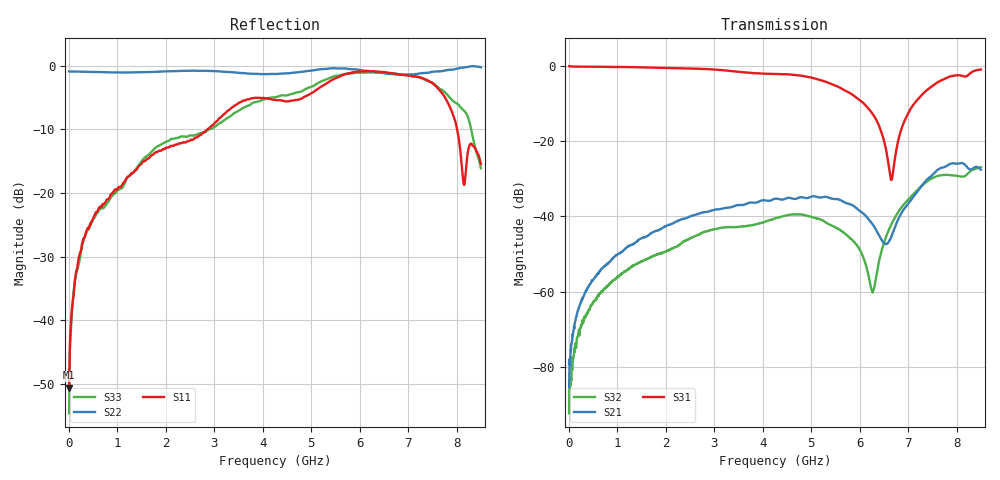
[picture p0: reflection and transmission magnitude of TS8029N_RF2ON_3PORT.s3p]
!Created with skrf (http://scikit-rf.org).
# GHz S RI R 50.0
!freq ReS11 ImS11 ReS12 ImS12 ReS13 ImS13
! ReS21 ImS21 ReS22 ImS22 ReS23 ImS23
! ReS31 ImS31 ReS32 ImS32 ReS33 ImS33
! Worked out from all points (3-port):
!   1601 points, 10 MHz to 8.5 GHz, reference 50 ohm
!   strongest paths, dB at 10 MHz, 2.132 GHz, 4.255 GHz, 6.378 GHz, 8.5 GHz:
!     S31: 0.0, -0.6, -2.1, -15.2, -0.9
!     S21: -85.2, -41.9, -35.3, -44.5, -27.5
!     S32: -92.3, -48.5, -40.5, -53.5, -26.9
!   lowest |S11| = -50.6 dB at 10 MHz (marker M1), VSWR 1.01, Z = 50 + j0.293 ohm
!   |S11| at or under -10 dB: start of sweep to 2.857 GHz; 8.01 GHz to end of sweep
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0.01  0.000466 0.00293  1.93e-05 5.24e-05  0.9945 -0.00837
      2.42e-05 4.9e-05  -0.9056 0.0034  3.17e-05 3.33e-05
      0.9947 -0.0084  2.39e-05 -3.76e-06  0.00165 0.00087
0.1426563  0.00914 -0.0205  8.28e-05 0.000425  0.9811 -0.0554
           7.62e-05 0.000413  -0.9016 0.0345  7.45e-05 -0.000171
           0.9813 -0.0553  5.38e-05 -0.000195  0.00638 -0.0209
0.6149125  -0.0033 -0.0751  -0.000115 0.00176  0.9498 -0.224
           -8.07e-05 0.00179  -0.8798 0.1527  -0.000539 -0.000703
           0.95 -0.2239  -0.000522 -0.00071  -0.00961 -0.0721
4.255  -0.5394 0.0344  0.00879 0.0148  -0.08 -0.7816
       0.00878 0.0148  -0.3182 0.802  -0.000224 0.00937
       -0.0812 -0.78  -0.00021 0.00944  -0.5661 -0.0107
5.634625  -0.5513 0.6351  0.014 0.00802  -0.36 -0.3438
          0.014 0.00801  -0.00423 0.9551  0.00468 0.00428
          -0.3603 -0.344  0.00467 0.00429  -0.5377 0.6626
6.266069  -0.2233 0.8805  0.00693 0.00373  -0.2108 -0.0966
          0.00696 0.00373  0.0242 0.9032  -0.000236 0.00098
          -0.211 -0.0966  -0.000203 0.000951  -0.3866 0.7992
6.653425  0.0469 0.8738  -0.0012 0.00525  -0.00276 -0.0304
          -0.00118 0.00525  0.1484 0.8496  -0.00746 0.00231
          -0.0029 -0.0304  -0.00749 0.00225  0.0808 0.8669
7.162825  0.4686 0.6786  -0.00785 0.0187  0.237 -0.2408
          -0.00786 0.0187  0.3716 0.778  -0.0137 0.0167
          0.237 -0.2409  -0.0136 0.0167  0.5839 0.5783
7.979988  0.3567 -0.017  0.0233 0.0447  0.000163 -0.7509
          0.0232 0.0446  0.5734 0.7522  0.0116 0.0329
          -0.000399 -0.75  0.0116 0.033  0.4543 0.2401
8.5  0.0927 0.1424  0.0237 0.0346  -0.2442 -0.8641
     0.0238 0.0346  0.5231 0.8232  0.0183 0.0413
     -0.2453 -0.8637  0.0182 0.0414  0.1547 -0.0269
